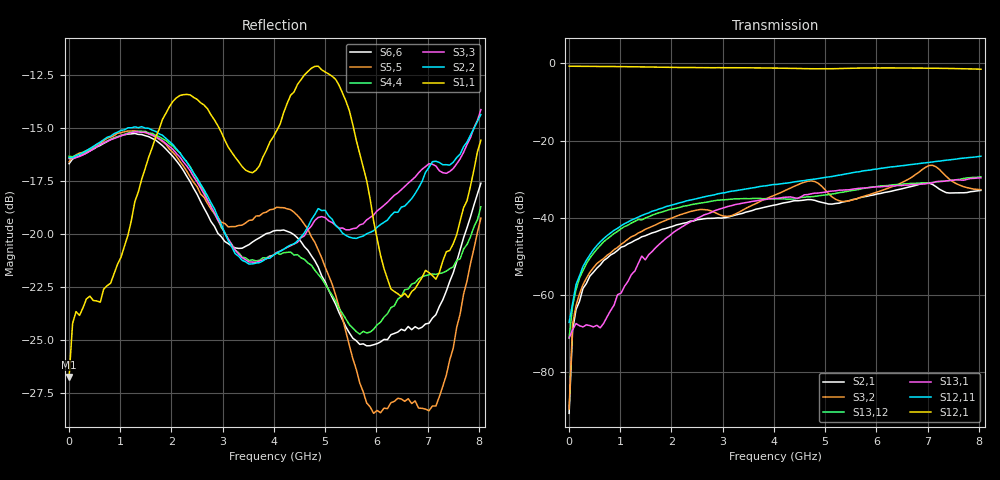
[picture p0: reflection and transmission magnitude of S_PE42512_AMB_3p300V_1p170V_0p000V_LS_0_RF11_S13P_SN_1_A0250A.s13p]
! Device ID: PE42512
! File Path: z:\PE42512\TE_GND_Post_Char_S-Param\All Parts\AMB\3p300\LS_0_RF11\PE42512_AMB_3p300V_1p170V_0p000V_LS_0_RF11_S13P_SN_1_A0250A.s13p
! Serial: 1
! Lot: A0250A
! Temp: AMB
! VDD: 3.300
! VSS: 0.000
! Control_Hi: 1.170
! Control_Lo: 0.000
! Logic State: LS_0_RF11
! Port 1:
! Port 2:
! Port 3:
! Port 4:
! Port 5:
! Port 6:
! Port 7:
! Port 8:
! Port 9:
! Port 10:
! Port 11:
! Port 12:
! Port 13:
! ThroughPath:1-12
! IDD: 0.0001072103
! ISS/IDD2: 5e-008
! IDMM3/IDD3: -1.952e-007
! Comment:
#  Hz  S  RI  R  50
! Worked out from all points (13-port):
!   120 points, 10 MHz to 8.037 GHz, reference 50 ohm
!   strongest paths, dB at 10 MHz, 2.034 GHz, 4.057 GHz, 6.08 GHz, 8.037 GHz:
!     S12,1: -0.7, -1.1, -1.2, -1.2, -1.5
!     S12,11: -67.1, -36.6, -31.4, -27.2, -24.1
!     S13,1: -71.1, -43.9, -35.0, -32.0, -29.7
!     S13,12: -71.1, -37.7, -35.1, -31.7, -29.4
!     S3,2: -89.5, -39.9, -33.9, -33.0, -32.7
!     S2,1: -90.6, -42.2, -36.6, -33.7, -32.9
!   lowest |S11| = -26.7 dB at 10 MHz (marker M1), VSWR 1.10, Z = 54.1 - j2.43 ohm
!   |S11| at or under -10 dB: start of sweep to end of sweep
